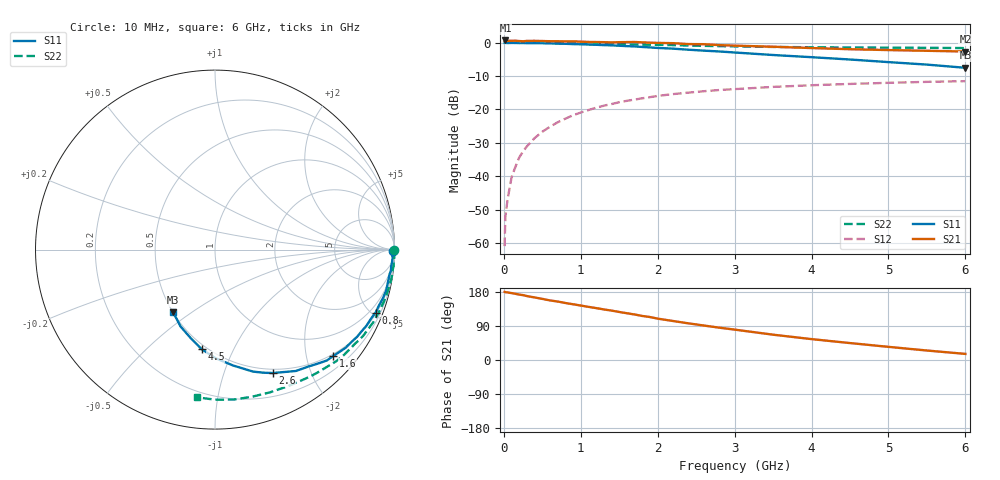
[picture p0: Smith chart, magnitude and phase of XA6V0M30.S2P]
! SIEMENS Discrete & RF Semiconductors
! BFY180
! Si NPN RF Bipolar Junction Transistor in MICRO-X
! VCE = 6 V  IC = 0.3 mA
! Common Emitter S-Parameters:  May  1997
# GHz  S  MA  R  50
!  f  S11  S21  S12  S22
! GHz  MAG  ANG  MAG  ANG  MAG  ANG  MAG  ANG
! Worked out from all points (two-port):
!   36 points, 10 MHz to 6 GHz, reference 50 ohm
!   highest |S21| = 0.65 dB at 20 MHz (marker M1); lowest = -2.7 dB at 6 GHz (marker M2)
!   |S21| within 3 dB of the highest: start of sweep to 5.284 GHz
!   lowest |S11| = -7.5 dB at 6 GHz (marker M3), VSWR 2.45, Z = 25.1 - j21.3 ohm
!   |S11| at or under -10 dB: nowhere
!   |S22| runs from -1.6 to 0.0 dB; largest |S21 - S12| = 1.1
!   S11 on the Smith chart (normalised r, x): 10 MHz: open; 800 MHz: 0.57, -5.23; 1.6 GHz: 0.46, -2.54; 2.6 GHz: 0.45, -1.47; 4.5 GHz: 0.47, -0.76; 6 GHz: 0.50, -0.43
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0.01  0.9905 -0.3  1.05 179.8  0.0009 87.3  0.9986 -0.2
0.02  0.9916 -0.7  1.078 179.0  0.0025 91.1  0.9999 -0.4
0.05  0.9863 -1.3  1.065 178.3  0.0046 89.7  1 -1.0
0.1  0.9907 -2.7  1.065 176.6  0.0096 89.7  0.9999 -2.0
0.2  0.9861 -5.3  1.057 172.6  0.0191 86.2  0.9978 -4.1
0.25  0.987 -6.9  1.049 171.2  0.0236 84.4  0.9999 -5.2
0.3  0.9822 -8.0  1.061 168.7  0.0281 83.6  0.9969 -6.1
0.4  0.9805 -10.8  1.064 165.1  0.0373 81.4  0.997 -8.3
0.6  0.9745 -15.9  1.05 157.2  0.0552 76.7  0.9921 -12.3
0.8  0.9612 -21.4  1.044 150.4  0.0729 72.4  0.986 -16.4
1.1  0.9354 -29.0  1.024 140.2  0.0979 65.5  0.9739 -22.4
1.6  0.8865 -41.9  1.019 123.4  0.1347 55.1  0.9481 -32.1
1.8  0.8616 -47.0  1.01 116.2  0.1471 51.3  0.9355 -35.7
2.2  0.8128 -56.3  0.982 102.9  0.1698 43.8  0.9178 -42.7
2.6  0.7587 -65.0  0.948 91.0  0.1874 37.2  0.8951 -49.1
2.8  0.7378 -68.4  0.918 85.3  0.1954 34.3  0.8866 -52.1
3.5  0.6531 -81.2  0.868 66.8  0.2176 24.6  0.8625 -62.0
4  0.6057 -89.6  0.83 55.1  0.2304 18.5  0.8523 -68.9
4.5  0.5592 -97.7  0.797 44.7  0.241 12.9  0.8455 -75.8
5  0.5112 -105.4  0.774 34.7  0.2504 7.6  0.842 -82.8
5.5  0.4691 -114.2  0.755 25.0  0.2589 2.3  0.8362 -89.9
6  0.4203 -123.6  0.736 16.1  0.2653 -3.3  0.8293 -97.1
